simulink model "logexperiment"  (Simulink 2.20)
settings: Solver=ode45  StartTime=0.0  StopTime=tstop  RelTol=1e-3  AbsTol=1e-6
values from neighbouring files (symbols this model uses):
  h = 0.05    [initlab3.m]
undefined symbols (not defined in the file or in its folder): Amp, N
libraries: simulink x1

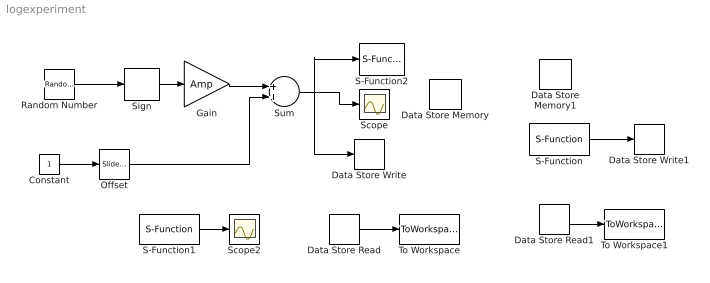
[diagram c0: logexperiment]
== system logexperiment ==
  Constant : Constant  Value=1
  Data Store Memory : DataStoreMemory  DataStoreName=logA  InitialValue=0
  Data Store Memory1 : DataStoreMemory  DataStoreName=logB  InitialValue=0
  Data Store Read : DataStoreRead  DataStoreName=logA  SampleTime=-1
  Data Store Read1 : DataStoreRead  DataStoreName=logB  SampleTime=-1
  Data Store Write : DataStoreWrite  DataStoreName=logA  SampleTime=h
  Data Store Write1 : DataStoreWrite  DataStoreName=logB  SampleTime=h
  Gain : Gain  Gain=Amp
  Offset : simulink/Linear/Slider Gain  low=-1  gain=0  high=1
  Random Number : RandomNumber  Mean=0  Variance=1  Seed=0  SampleTime=h*N
  S-Function : S-Function  FunctionName=analogin  Parameters=0  PortCounts=[]  SFunctionModules=''
  S-Function1 : S-Function  FunctionName=timer  Parameters=h  PortCounts=[]  SFunctionModules=''
  S-Function2 : S-Function  FunctionName=analogout  Parameters=0  PortCounts=[]  SFunctionModules=''
  Scope : Scope
  Scope2 : Scope
  Sign : Signum
  Sum : Sum  Inputs=++
  To Workspace : ToWorkspace  VariableName=u  SampleTime=-1
  To Workspace1 : ToWorkspace  VariableName=theta  SampleTime=-1
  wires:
  Random Number/1 -> Sign/1
  Sign/1 -> Gain/1
  Constant/1 -> Offset/1
  Gain/1 -> Sum/1
  Offset/1 -> Sum/2
  Sum/1 -> Scope/1, Data Store Write/1, S-Function2/1
  Data Store Read/1 -> To Workspace/1
  S-Function1/1 -> Scope2/1
  S-Function/1 -> Data Store Write1/1
  Data Store Read1/1 -> To Workspace1/1
